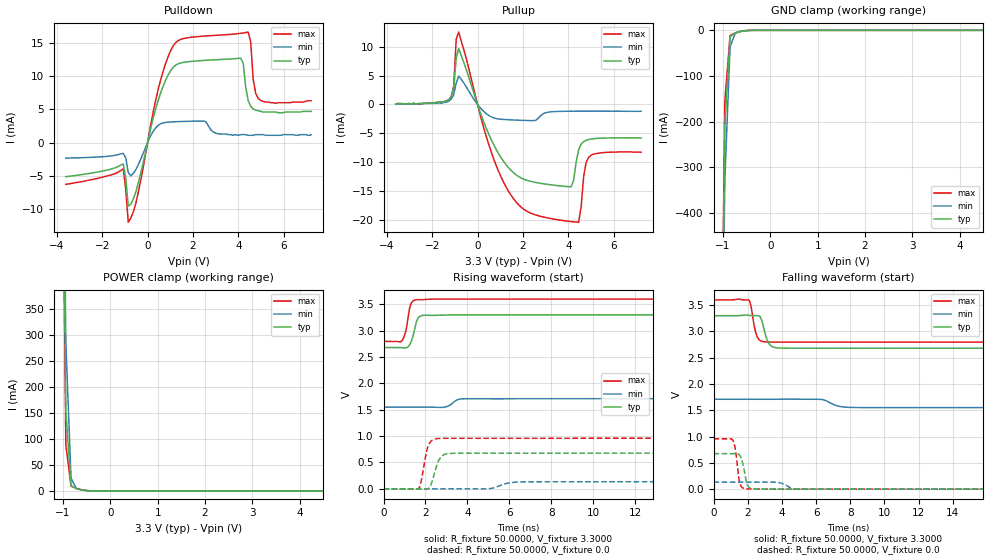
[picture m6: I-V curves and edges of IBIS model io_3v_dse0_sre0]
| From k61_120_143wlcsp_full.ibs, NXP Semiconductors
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[Model]  io_3v_dse0_sre0
|   Model io_3v_dse0_sre0
| Library cells for typ/min/max conditions are connected as defined below:
|  pad - External Pad
|  ipp_do_3v - Core Input
|  ipp_obe_3v - Output Buffer Enable
|  esd_boost - vdd_s_3v
|  esd_trigger - vss_s_3v
|  ipp_ame_3v - vss_s_3v
|  ipp_dse_3v - vss_s_3v
|  ipp_ina_3v - NC
|  ipp_ina_mux_3v - NC
|  ipp_ind_3v - NC
|  ipp_pue_3v - vss_s_3v
|  ipp_sre_3v - vss_s_3v
|  tie_3v - vdd_s_3v
|  tie_hi - vdd_s_lv
|  vbuf_3v - vdd_s_3v
|  vdd_s_3v - vdd_s_3v
|  vdd_s_lv - vdd_s_lv
|  vss_bulk - vss_s_3v
|  vss_s_3v - vss_s_3v
| All other pins connected to ground
Model_type I/O
Polarity   Non-Inverting
Enable   Active-High
Vinl =   1.1550V
Vinh =   2.3100V
Vmeas =  1.6500V
Cref =   25.0000pF
Rref =   50.0000
Vref =   0.0V
C_comp   1.9040pF   1.7928pF   2.1191pF
[Temperature Range]   25.0000   0.1250k   -40.0000
[Voltage Range]   3.3000V   1.7100V   3.6000V
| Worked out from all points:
|   slope of the pulldown table from 0 to 0.495 V, typ, clamps not added: 74.6 ohm
|   slope of the pullup table from 0 to 0.495 V, typ, clamps not added: 96.1 ohm
|   GND clamp passes 1 mA (typ) near -0.54 V on its own axis
|   POWER clamp passes 1 mA (typ) near -0.53 V on its own axis
|   rising waveform, R_fixture 50.0000, V_fixture 3.3000: 20-80 % time 244ps typ, 321ps min, 217ps max; typ from 2.68 V to 3.3 V
|   rising waveform, R_fixture 50.0000, V_fixture 0.0: 20-80 % time 323ps typ, 607ps min, 270ps max; typ from 0 V to 0.676 V
|   falling waveform, R_fixture 50.0000, V_fixture 3.3000: 20-80 % time 337ps typ, 645ps min, 278ps max; typ from 3.3 V to 2.68 V
|   falling waveform, R_fixture 50.0000, V_fixture 0.0: 20-80 % time 258ps typ, 475ps min, 218ps max; typ from 0.676 V to 0 V
[Pulldown]
|Voltage   I(typ)   I(min)   I(max)
-3.6V     -5.11mA    -2.33mA    -6.26mA
-1.07V    -3.221mA   -1.617mA   -3.914mA
-850mV    -9.536mA   -4.465mA   -11.95mA
-520mV    -7.435mA   -4.073mA   -9.159mA
580mV     7.513mA    2.844mA    9.475mA
1.46V     11.97mA    3.168mA    15.51mA
4.1V      12.68mA    1.2mA      16.42mA
4.43V     6.32mA     1.1mA      16.6mA
4.54V     5.46mA     1.1mA      15.13mA
4.65V     5.07mA     1.1mA      9.53mA
4.87V     4.8mA      1.2mA      6.66mA
7.2V      4.7mA      1.2mA      6.3mA
[Pullup]
|Voltage   I(typ)   I(min)   I(max)
-3.6V     100uA      0A         100uA
-1.27V    830uA      570uA      820uA
-1.05V    2.86mA     1.69mA     3.17mA
-940mV    8.013mA    3.699mA    11.33mA
-830mV    9.687mA    4.912mA    12.52mA
710mV     -6.946mA   -2.314mA   -9.402mA
2.14V     -13.06mA   -2.762mA   -18.39mA
4.12V     -14.22mA   -1.16mA    -20.25mA
4.45V     -7.839mA   -1.16mA    -20.35mA
4.67V     -6.422mA   -1.16mA    -12.47mA
4.89V     -6.059mA   -1.16mA    -9.139mA
7.2V      -5.79mA    -1.18mA    -8.25mA
[GND_clamp]
|Voltage   I(typ)   I(min)   I(max)
-3.6V     -47.78A    -47.06A    -48.3A
-1.07V    -1.101A    -1.183A    -1.105A
-960mV    -210.7mA   -326mA     -154mA
-850mV    -14.47mA   -36.11mA   -11.11mA
-740mV    -5.262mA   -6.034mA   -5.843mA
-520mV    -637uA     -915.4uA   -467.5uA
-300mV    -2.578uA   -18.09uA   -370.9nA
7.2V      0A         0A         0A
[POWER_clamp]
|Voltage   I(typ)   I(min)   I(max)
-3.6V     52.51A     51.88A     52.98A
-1.05V    1.126A     1.265A     1.065A
-940mV    154.2mA    286.1mA    88.03mA
-830mV    9.989mA    24.5mA     9.181mA
-720mV    4.227mA    4.408mA    5.116mA
-390mV    66.57uA    164uA      29.9uA
7.2V      0A         0A         0A
[Ramp]
| variable   typ   min   max
dV/dt_r  0.4057/0.3226n   80.3005m/0.6074n   0.5756/0.2700n
dV/dt_f  0.3715/0.3371n   95.3004m/0.6451n   0.4821/0.2777n
R_load = 50.0000
[Rising Waveform]
R_fixture= 50.0000
V_fixture= 3.3000
V_fixture_min= 1.7100
V_fixture_max= 3.6000
|time   V(typ)   V(min)   V(max)
0s        2.681V     1.551V     2.796V
899.8ps   2.677V     1.551V     2.822V
1.069ns   2.674V     1.551V     3.007V
1.285ns   2.765V     1.552V     3.484V
1.54ns    3.124V     1.552V     3.587V
1.671ns   3.249V     1.551V     3.589V
1.967ns   3.294V     1.551V     3.591V
2.989ns   3.299V     1.555V     3.6V
3.825ns   3.3V       1.708V     3.6V
20ns      3.3V       1.71V      3.6V
[Rising Waveform]
R_fixture= 50.0000
V_fixture= 0.0
V_fixture_min= 0.0
V_fixture_max= 0.0
|time   V(typ)   V(min)   V(max)
0s        5.331nV    455.6nV    4.026nV
1.674ns   -2.924mV   7.535uV    6.896mV
1.761ns   -1.492mV   9.343uV    81.95mV
2.013ns   -1.23mV    24.58uV    642.6mV
2.158ns   11.49mV    36.23uV    843.1mV
2.538ns   442.5mV    41.3uV     952.1mV
2.762ns   614.5mV    -50.52uV   956.9mV
3.292ns   673.5mV    -1.372mV   958.5mV
6.72ns    675.9mV    132.4mV    959mV
20ns      676.1mV    133.8mV    959.4mV
[Falling Waveform]
R_fixture= 50.0000
V_fixture= 3.3000
V_fixture_min= 1.7100
V_fixture_max= 3.6000
|time   V(typ)   V(min)   V(max)
0s        3.3V       1.71V      3.6V
2.061ns   3.307V     1.71V      3.599V
2.537ns   3.3V       1.71V      2.911V
2.725ns   3.283V     1.71V      2.83V
2.991ns   2.992V     1.71V      2.804V
3.271ns   2.756V     1.71V      2.8V
3.902ns   2.685V     1.711V     2.797V
6.335ns   2.681V     1.707V     2.797V
7.893ns   2.681V     1.557V     2.797V
20ns      2.681V     1.551V     2.796V
[Falling Waveform]
R_fixture= 50.0000
V_fixture= 0.0
V_fixture_min= 0.0
V_fixture_max= 0.0
|time   V(typ)   V(min)   V(max)
0s        676.3mV    133.9mV    959.6mV
1.117ns   677mV      133.9mV    938.4mV
1.259ns   677.9mV    133.8mV    798.4mV
1.536ns   640.6mV    133.8mV    120.1mV
1.837ns   278.8mV    133.8mV    8.012mV
2.019ns   57.67mV    133.8mV    4.125mV
2.364ns   3.713mV    133.9mV    3.367mV
3.83ns    333.2uV    125.8mV    395.8uV
4.967ns   258.4uV    1.134mV    353.4uV
20ns      96.45uV    25.87uV    133.2uV
